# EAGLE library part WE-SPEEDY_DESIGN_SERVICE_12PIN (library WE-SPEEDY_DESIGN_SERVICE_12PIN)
WE-Speedy Design Service, 12 Pin - Any application that fits package style - Switch Mode Power: Flyback, Forward, Push-Pull, Coupled Inductor -- Telecom Applications: xDSL, POTS Splitter Inductors
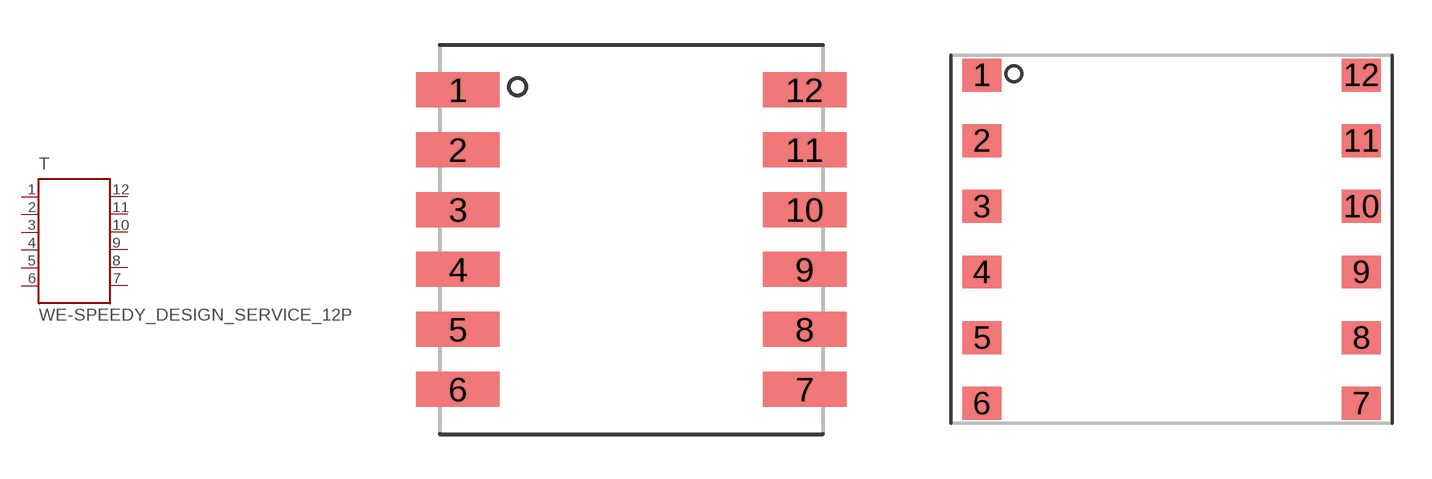
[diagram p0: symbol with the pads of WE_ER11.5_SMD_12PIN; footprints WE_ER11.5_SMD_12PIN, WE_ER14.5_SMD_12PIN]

Designator prefix T

## WE-SPEEDY_DESIGN_SERVICE_12PIN_ER11.5_SMD  [WE_ER11.5_SMD_12PIN]
1  1  pas
2  2  pas
3  3  pas
4  4  pas
5  5  pas
6  6  pas
7  7  pas
8  8  pas
9  9  pas
10  10  pas
11  11  pas
12  12  pas

## WE-SPEEDY_DESIGN_SERVICE_12PIN_ER14.5_SMD  [WE_ER14.5_SMD_12PIN]
Pads as for WE_ER11.5_SMD_12PIN

## WE-SPEEDY_DESIGN_SERVICE_12PIN_EFD15_SMD  [WE_EFD15_SMD_12PIN]
Pads as for WE_ER11.5_SMD_12PIN

## WE-SPEEDY_DESIGN_SERVICE_12PIN-750310617_EFD20_SMD (MPN: 750310617; OC_FARNELL: 1895759; OC_NEWARK: 47T5819; PACKAGE: EFD20_SMD_12PIN; SUPPLIER: Würth Elektronik eiSos GmbH), WE-SPEEDY_DESIGN_SERVICE_12PIN-750311385_EFD20_SMD (MPN: 750311385; OC_FARNELL: 1895757; OC_NEWARK: 47T5828; PACKAGE: EFD20_SMD_12PIN; SUPPLIER: Würth Elektronik eiSos GmbH), WE-SPEEDY_DESIGN_SERVICE_12PIN-750311597_EFD20_SMD (MPN: 750311597; OC_FARNELL: 1895761; OC_NEWARK: 47T5848; PACKAGE: EFD20_SMD_12PIN; SUPPLIER: Würth Elektronik eiSos GmbH), WE-SPEEDY_DESIGN_SERVICE_12PIN-750311598_EFD20_SMD (MPN: 750311598; OC_FARNELL: 1895762; OC_NEWARK: 47T5849; PACKAGE: EFD20_SMD_12PIN; SUPPLIER: Würth Elektronik eiSos GmbH), WE-SPEEDY_DESIGN_SERVICE_12PIN-750311599_EFD20_SMD (MPN: 750311599; OC_FARNELL: 1895763; OC_NEWARK: 47T5850; PACKAGE: EFD20_SMD_12PIN; SUPPLIER: Würth Elektronik eiSos GmbH), WE-SPEEDY_DESIGN_SERVICE_12PIN-750311600_EFD20_SMD (MPN: 750311600; OC_FARNELL: 1895764; OC_NEWARK: unknown; PACKAGE: EFD20_SMD_12PIN; SUPPLIER: Würth Elektronik eiSos GmbH), WE-SPEEDY_DESIGN_SERVICE_12PIN-750311604_EFD20_SMD (MPN: 750311604; OC_FARNELL: 1895765; OC_NEWARK: 47T5852; PACKAGE: EFD20_SMD_12PIN; SUPPLIER: Würth Elektronik eiSos GmbH), WE-SPEEDY_DESIGN_SERVICE_12PIN-750311605_EFD20_SMD (MPN: 750311605; OC_FARNELL: 1895766; OC_NEWARK: 47T5853; PACKAGE: EFD20_SMD_12PIN; SUPPLIER: Würth Elektronik eiSos GmbH), WE-SPEEDY_DESIGN_SERVICE_12PIN-750311607_EFD20_SMD (MPN: 750311607; OC_FARNELL: 1895767; OC_NEWARK: 47T5854; PACKAGE: EFD20_SMD_12PIN; SUPPLIER: Würth Elektronik eiSos GmbH), WE-SPEEDY_DESIGN_SERVICE_12PIN-750311608_EFD20_SMD (MPN: 750311608; OC_FARNELL: 1895768; OC_NEWARK: 47T5855; PACKAGE: EFD20_SMD_12PIN; SUPPLIER: Würth Elektronik eiSos GmbH), WE-SPEEDY_DESIGN_SERVICE_12PIN-750311797_EFD20_SMD (MPN: 750311797; OC_FARNELL: 1895769; OC_NEWARK: 47T5865; PACKAGE: EFD20_SMD_12PIN; SUPPLIER: Würth Elektronik eiSos GmbH)  [WE_EFD20_SMD_12PIN]
Pads as for WE_ER11.5_SMD_12PIN

## WE-SPEEDY_DESIGN_SERVICE_12PIN-750310988_EFD25_SMD (MPN: 750310988; OC_FARNELL: 1895780; OC_NEWARK: 47T5820; PACKAGE: EFD25-SMD; SUPPLIER: Würth Elektronik eiSos GmbH), WE-SPEEDY_DESIGN_SERVICE_12PIN-750311589_EFD25_SMD (MPN: 750311589; OC_FARNELL: 1895770; OC_NEWARK: 47T5840; PACKAGE: EFD25-SMD; SUPPLIER: Würth Elektronik eiSos GmbH), WE-SPEEDY_DESIGN_SERVICE_12PIN-750311590_EFD25_SMD (MPN: 750311590; OC_FARNELL: 1895772; OC_NEWARK: 47T5841; PACKAGE: EFD25-SMD; SUPPLIER: Würth Elektronik eiSos GmbH), WE-SPEEDY_DESIGN_SERVICE_12PIN-750311591_EFD25_SMD (MPN: 750311591; OC_FARNELL: 1895773; OC_NEWARK: 47T5842; PACKAGE: EFD25-SMD; SUPPLIER: Würth Elektronik eiSos GmbH), WE-SPEEDY_DESIGN_SERVICE_12PIN-750311592_EFD25_SMD (MPN: 750311592; OC_FARNELL: 1895774; OC_NEWARK: 47T5843; PACKAGE: EFD25-SMD; SUPPLIER: Würth Elektronik eiSos GmbH), WE-SPEEDY_DESIGN_SERVICE_12PIN-750311593_EFD25_SMD (MPN: 750311593; OC_FARNELL: 1895775; OC_NEWARK: 47T5844; PACKAGE: EFD25-SMD; SUPPLIER: Würth Elektronik eiSos GmbH), WE-SPEEDY_DESIGN_SERVICE_12PIN-750311594_EFD25_SMD (MPN: 750311594; OC_FARNELL: 1895776; OC_NEWARK: 47T5845; PACKAGE: EFD25-SMD; SUPPLIER: Würth Elektronik eiSos GmbH), WE-SPEEDY_DESIGN_SERVICE_12PIN-750311595_EFD25_SMD (MPN: 750311595; OC_FARNELL: 1895777; OC_NEWARK: 47T5846; PACKAGE: EFD25-SMD; SUPPLIER: Würth Elektronik eiSos GmbH), WE-SPEEDY_DESIGN_SERVICE_12PIN-750311596_EFD25_SMD (MPN: 750311596; OC_FARNELL: 1895778; OC_NEWARK: 47T5847; PACKAGE: EFD25-SMD; SUPPLIER: Würth Elektronik eiSos GmbH), WE-SPEEDY_DESIGN_SERVICE_12PIN-750311771_EFD25_SMD (MPN: 750311771; OC_FARNELL: 1895779; OC_NEWARK: 47T5863; PACKAGE: EFD25-SMD; SUPPLIER: Würth Elektronik eiSos GmbH), WE-SPEEDY_DESIGN_SERVICE_12PIN-750311783_EFD25_SMD (MPN: 750311783; OC_FARNELL: 1895781; OC_NEWARK: 47T5864; PACKAGE: EFD25-SMD; SUPPLIER: Würth Elektronik eiSos GmbH), WE-SPEEDY_DESIGN_SERVICE_12PIN-750311889_EFD25_SMD (MPN: 750311889; OC_FARNELL: 1895731; OC_NEWARK: 47T5867; PACKAGE: EFD25-SMD; SUPPLIER: Würth Elektronik eiSos GmbH)  [WE_EFD25_SMD_12PIN]
Pads as for WE_ER11.5_SMD_12PIN

## WE-SPEEDY_DESIGN_SERVICE_12PIN_ER28_THT  [WE_ER28_THT_HORIZONTAL_12PIN]
Pads as for WE_ER11.5_SMD_12PIN

## Footprint WE_ER11.5_SMD_12PIN (pad centres in mm)
Transformer, ER11.5 SMD 12 Pin
smd 2.79 x 1.17: 1 -5.79,5; 2 -5.79,3; 3 -5.79,1; 4 -5.79,-1; 5 -5.79,-3; 6 -5.79,-5; 7 5.79,-5; 8 5.79,-3; 9 5.79,-1; 10 5.79,1; 11 5.79,3; 12 5.79,5

## Footprint WE_ER14.5_SMD_12PIN (pad centres in mm)
Transformer, ER14.5 SMD 12 Pin
smd 1.5 x 1.25: 1 -7.225,6.25; 2 -7.225,3.75; 3 -7.225,1.25; 4 -7.225,-1.25; 5 -7.225,-3.75; 6 -7.225,-6.25; 7 7.225,-6.25; 8 7.225,-3.75; 9 7.225,-1.25; 10 7.225,1.25; 11 7.225,3.75; 12 7.225,6.25

## Footprint WE_EFD15_SMD_12PIN (pad centres in mm)
Transformer, EFD15 SMD 12 Pin
smd 2.62 x 1.17: 1 -9.895,6.225; 2 -9.895,3.735; 3 -9.895,1.245; 4 -9.895,-1.245; 5 -9.895,-3.735; 6 -9.895,-6.225; 7 9.895,-6.225; 8 9.895,-3.735; 9 9.895,-1.245; 10 9.895,1.245; 11 9.895,3.735; 12 9.895,6.225

## Footprint WE_EFD20_SMD_12PIN (pad centres in mm)
Transformer, EFD20 SMD 12 Pin
smd 3.05 x 1.27: 1 -13.26,7.5; 2 -13.26,4.5; 3 -13.26,1.5; 4 -13.26,-1.5; 5 -13.26,-4.5; 6 -13.26,-7.5; 7 13.26,-7.5; 8 13.26,-4.5; 9 13.26,-1.5; 10 13.26,1.5; 11 13.26,4.5; 12 13.26,7.5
